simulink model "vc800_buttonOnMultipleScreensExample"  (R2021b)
settings: Solver=FixedStepDiscrete  StartTime=0.0  StopTime=10.0  FixedStep=0.01  RelTol=1e-3  EnableMultiTasking=on
PreLoadFcn:
  | try, model_open; catch, disp('Error occurred while executing model pre-load callback: model_open.m'); disp('Please assure that the MATLAB working directory is set to the model directory before opening.'); end
InitFcn:
  | try, model_open; catch, end
model workspace (MAT data in the model file):
  IOScreen_Label_XCoord = 1
  IOScreen_Row1_YCoord = 1
  IOScreen_Row2_YCoord = 12
  IOScreen_Value_XCoord = 110
  MainScreen_Row1_YCoord = 7
  MainScreen_Row2_YCoord = 23
  MainScreen_Symbols_XCoord = 1
  MainScreen_Units_XCoord = 69
  MainScreen_Value_XCoord = 64
undefined symbols (not defined in the file or in its folder): case, curr_screen, default, DISP, filtering, gesture, hex2dec, Mode, No, raptor_get_buildNum, raptor_get_safe_string, raptor_hwexp, raptor_xcp_function, Screens, VC800, Voltage
libraries: Raptor_display_lib x190, Raptor_lib x97, simulink_extras x11, Raptor_Datalogging_lib x10, simulink x2
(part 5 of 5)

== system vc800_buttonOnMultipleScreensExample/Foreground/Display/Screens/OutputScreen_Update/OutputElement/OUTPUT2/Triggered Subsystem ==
  Trigger : TriggerPort  VariantControl=Variant
  Constant2 : Constant
  D Latch : simulink_extras/Flip Flops/D Latch
  Unit Delay : UnitDelay  InitialCondition=InitialCondition  SampleTime=-1  HasFrameUpgradeWarning=on
  Out1 : Outport  VectorParamsAs1DForOutWhenUnconnected=off
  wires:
  Constant2/1 -> D Latch/2
  D Latch/1 -> Out1/1
  Unit Delay/1 -> D Latch/1
  D Latch/2 -> Unit Delay/1

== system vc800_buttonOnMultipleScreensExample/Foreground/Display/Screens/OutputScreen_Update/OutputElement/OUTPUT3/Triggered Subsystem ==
  Trigger : TriggerPort  VariantControl=Variant
  Constant2 : Constant
  D Latch : simulink_extras/Flip Flops/D Latch
  Unit Delay : UnitDelay  InitialCondition=InitialCondition  SampleTime=-1  HasFrameUpgradeWarning=on
  Out1 : Outport  VectorParamsAs1DForOutWhenUnconnected=off
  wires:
  D Latch/2 -> Unit Delay/1
  Unit Delay/1 -> D Latch/1
  D Latch/1 -> Out1/1
  Constant2/1 -> D Latch/2

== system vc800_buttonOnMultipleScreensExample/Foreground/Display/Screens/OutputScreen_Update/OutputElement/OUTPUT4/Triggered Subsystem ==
  Trigger : TriggerPort  VariantControl=Variant
  Constant2 : Constant
  D Latch : simulink_extras/Flip Flops/D Latch
  Unit Delay : UnitDelay  InitialCondition=InitialCondition  SampleTime=-1  HasFrameUpgradeWarning=on
  Out1 : Outport  VectorParamsAs1DForOutWhenUnconnected=off
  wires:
  Constant2/1 -> D Latch/2
  D Latch/1 -> Out1/1
  Unit Delay/1 -> D Latch/1
  D Latch/2 -> Unit Delay/1

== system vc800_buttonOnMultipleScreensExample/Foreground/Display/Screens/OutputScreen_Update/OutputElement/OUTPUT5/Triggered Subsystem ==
  Trigger : TriggerPort  VariantControl=Variant
  Constant2 : Constant
  D Latch : simulink_extras/Flip Flops/D Latch
  Unit Delay : UnitDelay  InitialCondition=InitialCondition  SampleTime=-1  HasFrameUpgradeWarning=on
  Out1 : Outport  VectorParamsAs1DForOutWhenUnconnected=off
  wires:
  D Latch/2 -> Unit Delay/1
  Unit Delay/1 -> D Latch/1
  D Latch/1 -> Out1/1
  Constant2/1 -> D Latch/2

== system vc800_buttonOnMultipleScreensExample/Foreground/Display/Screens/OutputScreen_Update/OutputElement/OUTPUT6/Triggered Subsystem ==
  Trigger : TriggerPort  VariantControl=Variant
  Constant2 : Constant
  D Latch : simulink_extras/Flip Flops/D Latch
  Unit Delay : UnitDelay  InitialCondition=InitialCondition  SampleTime=-1  HasFrameUpgradeWarning=on
  Out1 : Outport  VectorParamsAs1DForOutWhenUnconnected=off
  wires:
  Constant2/1 -> D Latch/2
  D Latch/1 -> Out1/1
  Unit Delay/1 -> D Latch/1
  D Latch/2 -> Unit Delay/1

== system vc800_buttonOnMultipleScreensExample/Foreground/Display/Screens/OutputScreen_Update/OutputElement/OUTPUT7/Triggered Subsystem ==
  Trigger : TriggerPort  VariantControl=Variant
  Constant2 : Constant
  D Latch : simulink_extras/Flip Flops/D Latch
  Unit Delay : UnitDelay  InitialCondition=InitialCondition  SampleTime=-1  HasFrameUpgradeWarning=on
  Out1 : Outport  VectorParamsAs1DForOutWhenUnconnected=off
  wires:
  D Latch/2 -> Unit Delay/1
  Unit Delay/1 -> D Latch/1
  D Latch/1 -> Out1/1
  Constant2/1 -> D Latch/2

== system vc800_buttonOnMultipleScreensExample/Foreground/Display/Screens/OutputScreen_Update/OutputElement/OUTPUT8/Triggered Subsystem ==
  Trigger : TriggerPort  VariantControl=Variant
  Constant2 : Constant
  D Latch : simulink_extras/Flip Flops/D Latch
  Unit Delay : UnitDelay  InitialCondition=InitialCondition  SampleTime=-1  HasFrameUpgradeWarning=on
  Out1 : Outport  VectorParamsAs1DForOutWhenUnconnected=off
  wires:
  Constant2/1 -> D Latch/2
  D Latch/1 -> Out1/1
  Unit Delay/1 -> D Latch/1
  D Latch/2 -> Unit Delay/1
